FUNCTION FC 16 : VOID
TITLE =ESPOSITO ANTONIO ANIELLO
AUTHOR : Esposito
FAMILY : EGAL_srl
NAME : WG_SOFT
VERSION : 0.1


VAR_TEMP
  Count_relax : INT ;
END_VAR
BEGIN
NETWORK
TITLE =WGSOFT "THE RELAX"

      U     M      1.0;
      U     M    255.5;
      FP    M     70.7;
      ZV    Z     10;
      BLD   101;
      U     M      1.0;
      L     C#60;
      S     Z     10;
      U     M     70.6;
      R     Z     10;
      L     Z     10;
      T     #Count_relax;
      NOP   0;
      NOP   0;
NETWORK
TITLE =WGSOFT "THE RELAX"
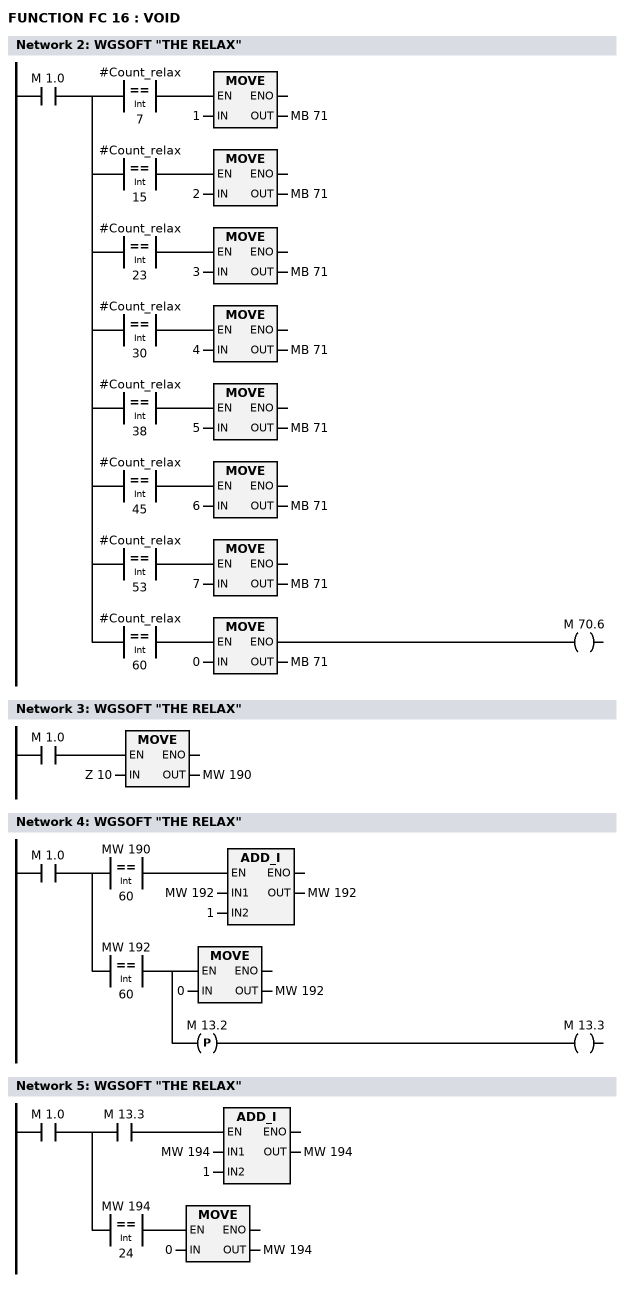
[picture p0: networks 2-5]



      U     M      1.0;
      =     L      2.0;
      U     L      2.0;
      U(    ;
      L     #Count_relax;
      L     7;
      ==I   ;
      )     ;
      SPBNB _001;
      L     1;
      T     MB    71;
_001: NOP   0;
      U     L      2.0;
      U(    ;
      L     #Count_relax;
      L     15;
      ==I   ;
      )     ;
      SPBNB _002;
      L     2;
      T     MB    71;
_002: NOP   0;
      U     L      2.0;
      U(    ;
      L     #Count_relax;
      L     23;
      ==I   ;
      )     ;
      SPBNB _003;
      L     3;
      T     MB    71;
_003: NOP   0;
      U     L      2.0;
      U(    ;
      L     #Count_relax;
      L     30;
      ==I   ;
      )     ;
      SPBNB _004;
      L     4;
      T     MB    71;
_004: NOP   0;
      U     L      2.0;
      U(    ;
      L     #Count_relax;
      L     38;
      ==I   ;
      )     ;
      SPBNB _005;
      L     5;
      T     MB    71;
_005: NOP   0;
      U     L      2.0;
      U(    ;
      L     #Count_relax;
      L     45;
      ==I   ;
      )     ;
      SPBNB _006;
      L     6;
      T     MB    71;
_006: NOP   0;
      U     L      2.0;
      U(    ;
      L     #Count_relax;
      L     53;
      ==I   ;
      )     ;
      SPBNB _007;
      L     7;
      T     MB    71;
_007: NOP   0;
      U     L      2.0;
      U(    ;
      L     #Count_relax;
      L     60;
      ==I   ;
      )     ;
      SPBNB _008;
      L     0;
      T     MB    71;
      SET   ;
      SAVE  ;
      CLR   ;
_008: U     BIE;
      =     M     70.6;
NETWORK
TITLE =WGSOFT "THE RELAX"

      U     M      1.0;
      SPBNB _009;
      L     Z     10;
      T     MW   190;
_009: NOP   0;
NETWORK
TITLE =WGSOFT "THE RELAX"

      U     M      1.0;
      =     L      2.0;
      U     L      2.0;
      U(    ;
      L     MW   190;
      L     60;
      ==I   ;
      )     ;
      SPBNB _00a;
      L     MW   192;
      L     1;
      +I    ;
      T     MW   192;
_00a: NOP   0;
      U     L      2.0;
      U(    ;
      L     MW   192;
      L     60;
      ==I   ;
      )     ;
      =     L      2.1;
      U     L      2.1;
      SPBNB _00b;
      L     0;
      T     MW   192;
_00b: NOP   0;
      U     L      2.1;
      FP    M     13.2;
      =     M     13.3;
NETWORK
TITLE =WGSOFT "THE RELAX"

      U     M      1.0;
      =     L      2.0;
      U     L      2.0;
      U     M     13.3;
      SPBNB _00c;
      L     MW   194;
      L     1;
      +I    ;
      T     MW   194;
_00c: NOP   0;
      U     L      2.0;
      U(    ;
      L     MW   194;
      L     24;
      ==I   ;
      )     ;
      SPBNB _00d;
      L     0;
      T     MW   194;
_00d: NOP   0;
END_FUNCTION

